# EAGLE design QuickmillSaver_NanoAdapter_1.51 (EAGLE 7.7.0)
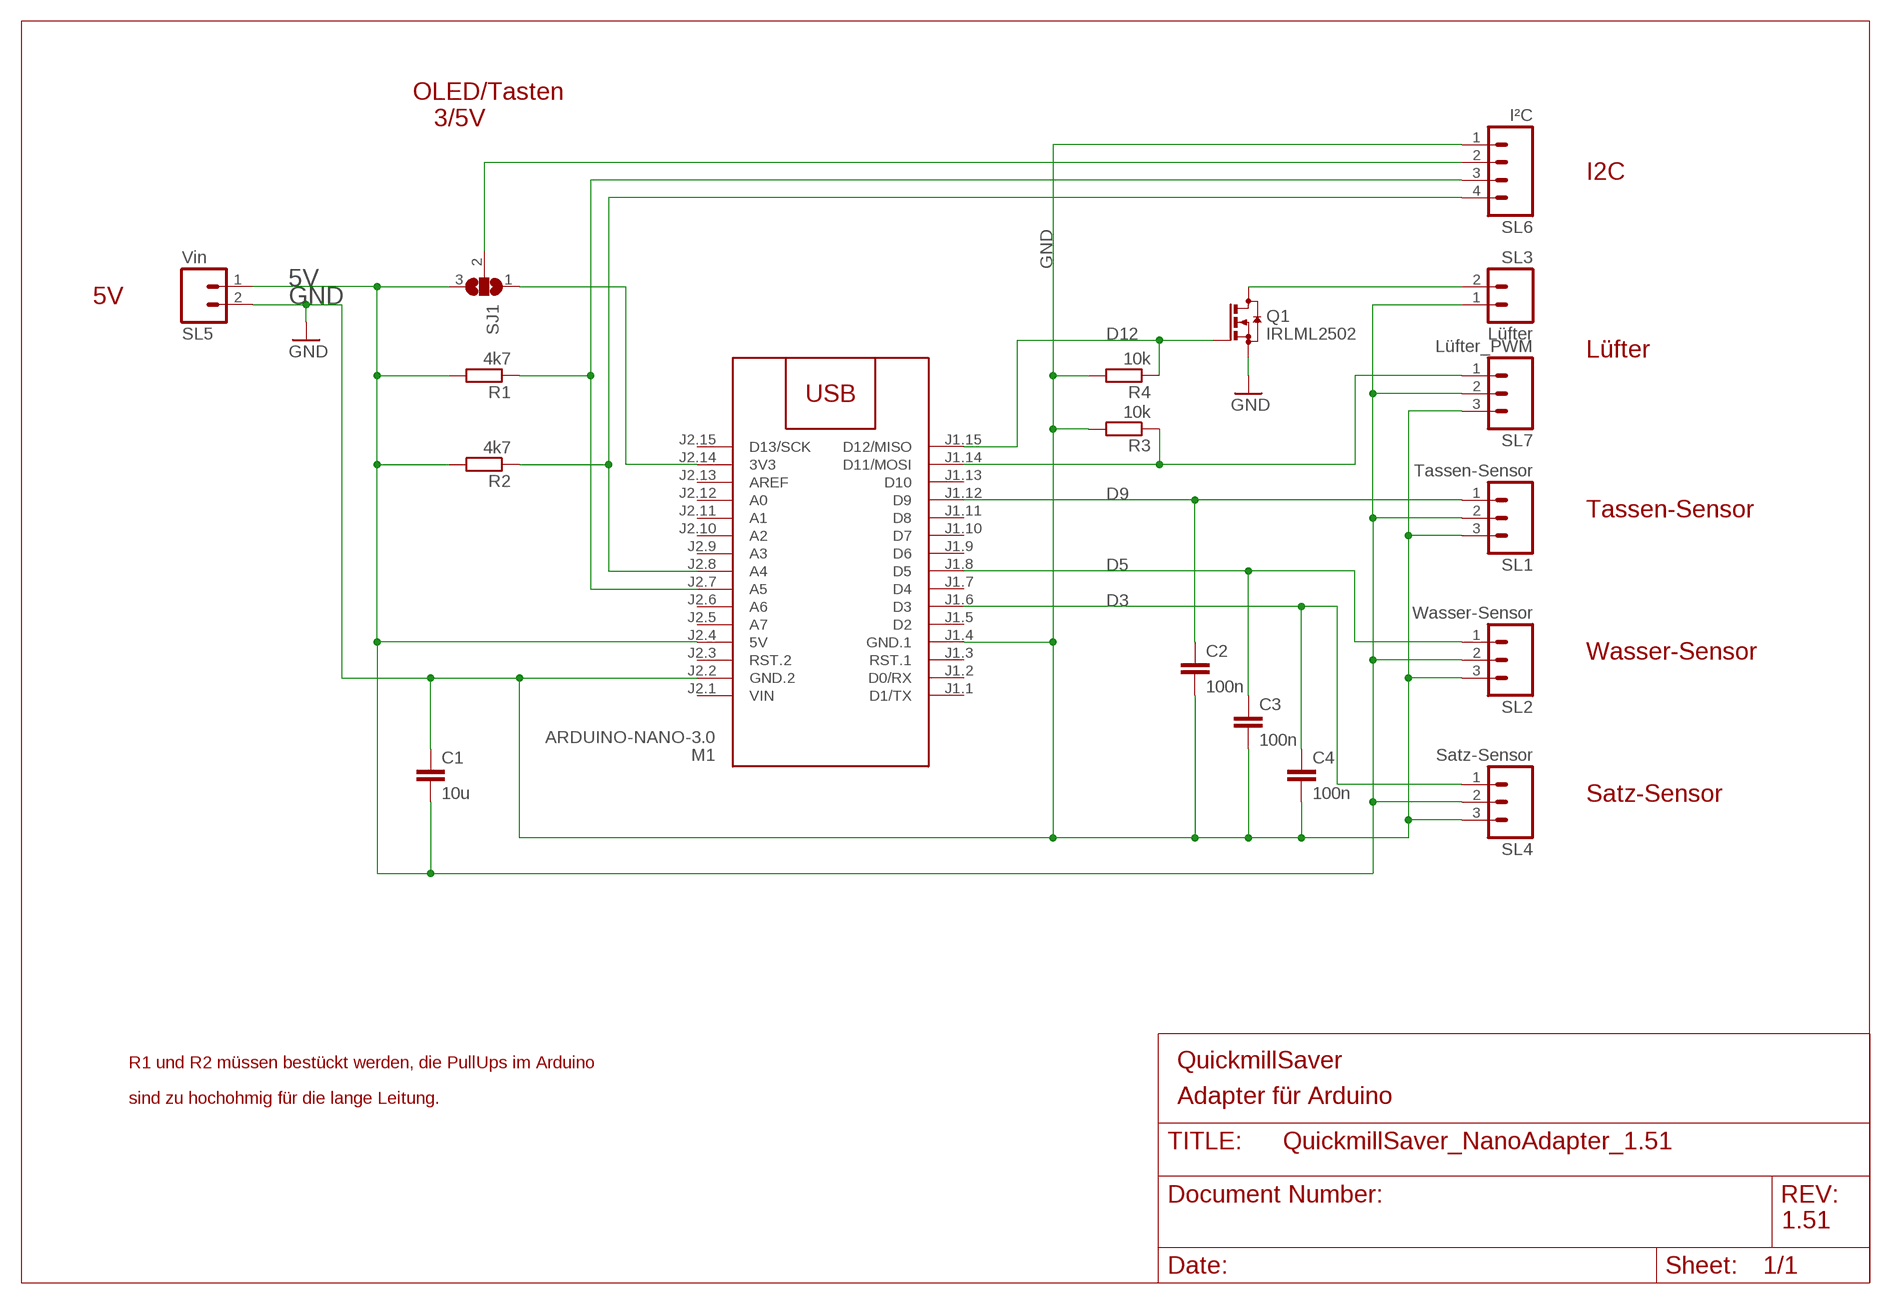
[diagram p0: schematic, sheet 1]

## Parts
C1  10u  C-EUC0805  [C0805]
C2  100n  C-EUC0603  [C0603]
C3  100n  C-EUC0603  [C0603]
C4  100n  C-EUC0603  [C0603]
M1  ARDUINO-NANO-3.0  [ARDUINO-NANO-3.0]
Q1  IRLML2502  BSS123  [SOT23]
R1  4k7  R-EU_R0603  [R0603]
R2  4k7  R-EU_R0603  [R0603]
R3  10k  R-EU_R0603  [R0603]
R4  10k  R-EU_R0603  [R0603]
SJ1  SJ2WW  [SJ_2W]
SL1  Tassen-Sensor  M03  [03P]
SL2  Wasser-Sensor  M03  [03P]
SL3  Lüfter  M02  [02P]
SL4  Satz-Sensor  M03  [03P]
SL5  Vin  M02  [02P]
SL6  I²C  M04  [04P]
SL7  Lüfter_PWM  M03  [03P]

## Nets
5V: C1.2 M1.J2.4(5V) R1.2 R2.2 SJ1.3 SL1.2 SL2.2 SL3.1 SL4.2 SL5.1 SL7.2
D3: C4.1 M1.J1.6(D3) SL4.1
D5: C3.1 M1.J1.8(D5) SL2.1
D9: C2.1 M1.J1.12(D9) SL1.1
D12: M1.J1.15(D12/MISO) Q1.1(G) R4.1
GND: C1.1 C2.2 C3.2 C4.2 M1.J1.4(GND.1) M1.J2.2(GND.2) Q1.2(S) R3.2 R4.2 SL1.3 SL2.3 SL4.3 SL5.2 SL6.1 SL7.3
N$1: M1.J2.14(3V3) SJ1.1
N$2: M1.J1.14(D11/MOSI) R3.1 SL7.1
N$3: Q1.3(D) SL3.2
N$9: SJ1.2 SL6.2
N$10: M1.J2.7(A5) R1.1 SL6.3
N$11: M1.J2.8(A4) R2.1 SL6.4
Unconnected: M1.J1.1(D1/TX) M1.J1.2(D0/RX) M1.J1.3(RST.1) M1.J1.5(D2) M1.J1.7(D4) M1.J1.9(D6) M1.J1.10(D7) M1.J1.11(D8) M1.J1.13(D10) M1.J2.3(RST.2) M1.J2.5(A7) M1.J2.6(A6) M1.J2.9(A3) M1.J2.10(A2) M1.J2.11(A1) M1.J2.12(A0) M1.J2.13(AREF) M1.J2.15(D13/SCK)

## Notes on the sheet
- OLED/Tasten
     3/5V
- I2C
- 5V
- Lüfter
- Tassen-Sensor
- Wasser-Sensor
- Satz-Sensor
- R1 und R2 müssen bestückt werden, die PullUps im Arduino | QuickmillSaver
- sind zu hochohmig für die lange Leitung. | Adapter für Arduino
- 1.51

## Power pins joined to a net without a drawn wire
VIN: M1.J2.1(VIN)

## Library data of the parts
C1-C4 = rcl:C-EU: CAPACITOR, European symbol
M1 = diy-modules:ARDUINO-NANO-3.0: Arduino Nano 3.0 and compatible devices More details available here: https://www.arduino.cc/en/Main/ArduinoBoardNano Click here to find device on ebay.com
Q1 = transistor-small-signal:BSS123: N-CHANNEL MOS FET
R1-R4 = rcl:R-EU_: RESISTOR, European symbol
SJ1 = jumper:SJ2W: SMD solder JUMPER
SL1 SL2 SL4 SL7 = con-amp-quick:M03: AMP QUICK CONNECTOR
SL3 SL5 = con-amp-quick:M02: AMP QUICK CONNECTOR
SL6 = con-amp-quick:M04: AMP QUICK CONNECTOR

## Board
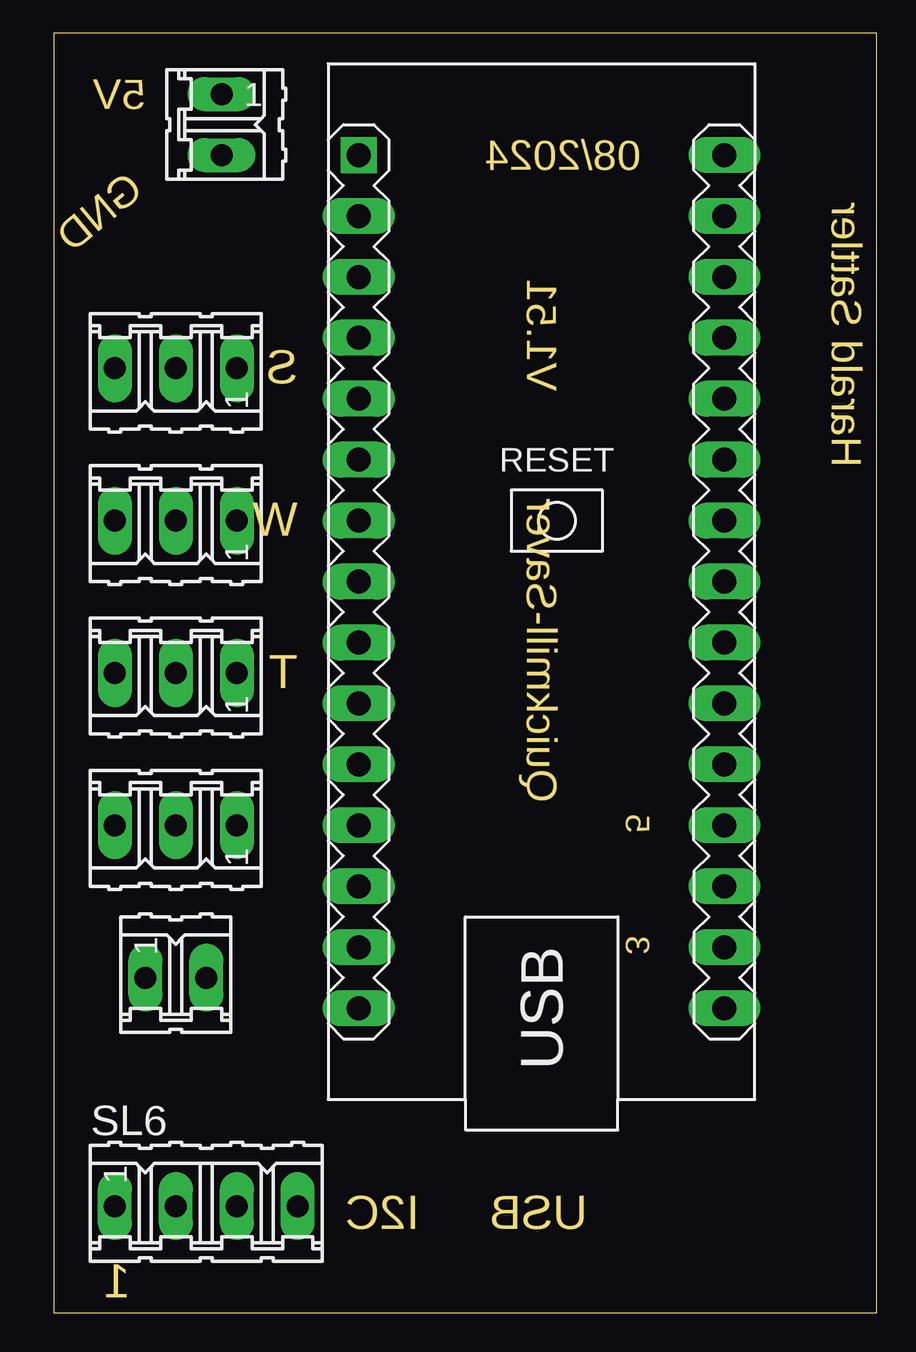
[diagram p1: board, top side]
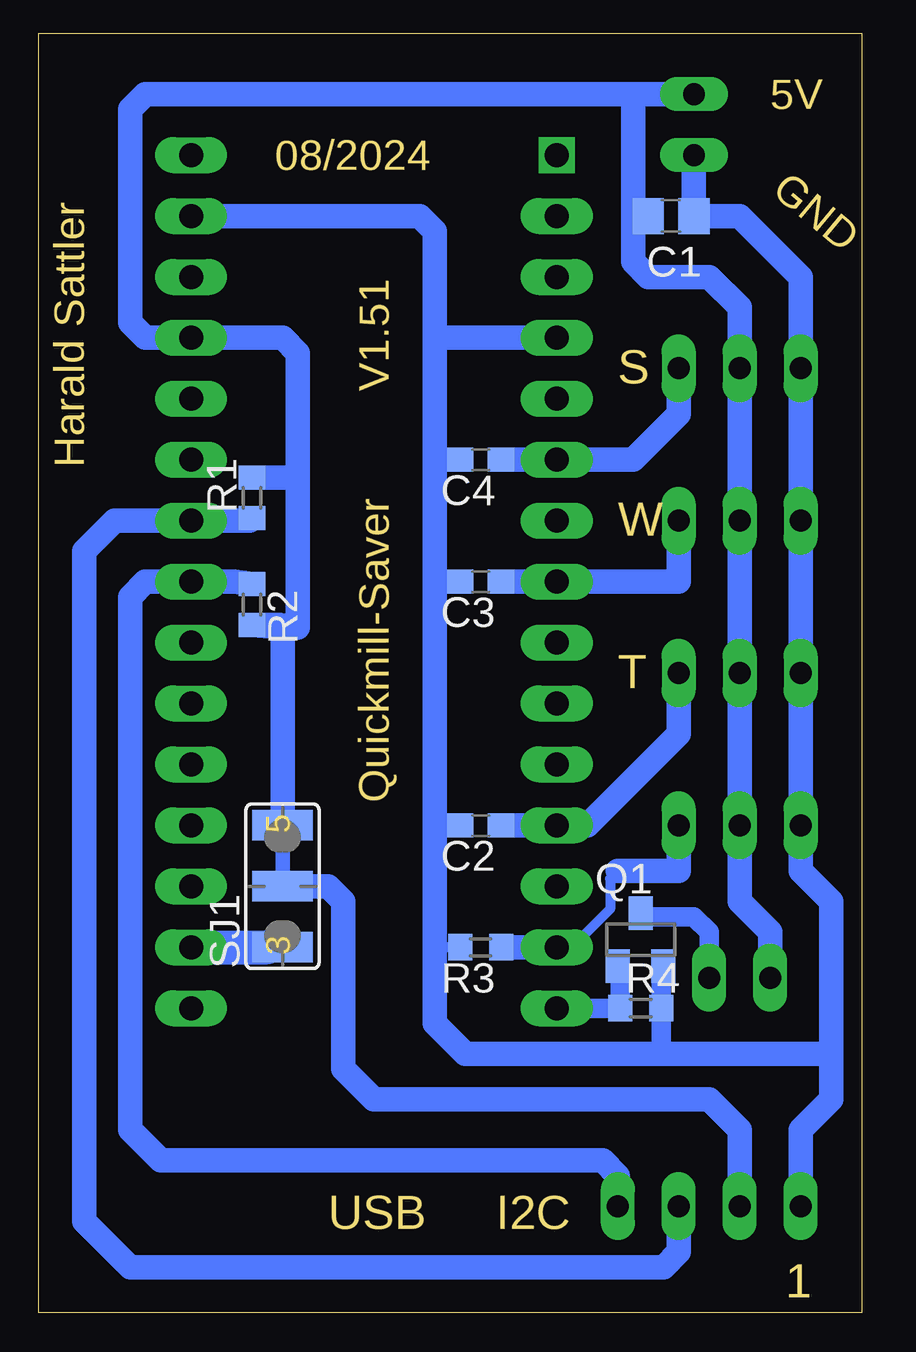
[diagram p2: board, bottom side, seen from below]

No outline drawn. Coordinates in mm, seen from the top.
Copper layers (1*16): Top 0.035mm / dielectric 1.5mm / Bottom 0.035mm
Design rules "default *": minimum track width 10mil, minimum drill 24mil, track to track 0.3mm, track to pad 0.3mm, pad to pad 0.3mm, via to via 0.3mm, smd to smd 0.3mm, copper to edge 40mil, drill to drill 8mil, minimum pad ring 10mil, minimum via ring 8mil, stop-mask expansion 4mil, vias tented up to drill 0mil, thermal gap 10mil
Milling: 4 lines

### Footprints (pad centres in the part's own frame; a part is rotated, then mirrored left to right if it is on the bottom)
C0805 = smd 1.3 x 1.5: 1 -0.95,0; 2 0.95,0
C0603 = smd 1.1 x 1: 1 -0.85,0; 2 0.85,0
ARDUINO-NANO-3.0 = drill 1 pad 1.27 square: J1.1 17.78,7.62 | drill 1 pad 1.27 long: J1.2 15.24,7.62; J1.3 12.7,7.62; J1.4 10.16,7.62; J1.5 7.62,7.62; J1.6 5.08,7.62; J1.7 2.54,7.62; J1.8 0,7.62; J1.9 -2.54,7.62; J1.10 -5.08,7.62; J1.11 -7.62,7.62; J1.12 -10.16,7.62; J1.13 -12.7,7.62; J1.14 -15.24,7.62; J1.15 -17.78,7.62; J2.1 17.78,-7.62; J2.2 15.24,-7.62; J2.3 12.7,-7.62; J2.4 10.16,-7.62; J2.5 7.62,-7.62; J2.6 5.08,-7.62; J2.7 2.54,-7.62; J2.8 0,-7.62; J2.9 -2.54,-7.62; J2.10 -5.08,-7.62; J2.11 -7.62,-7.62; J2.12 -10.16,-7.62; J2.13 -12.7,-7.62; J2.14 -15.24,-7.62; J2.15 -17.78,-7.62
SOT23 = smd 1 x 1.4: 1 -0.95,-1.1; 2 0.95,-1.1; 3 0,1.1
R0603 = smd 1 x 1.1: 1 -0.85,0; 2 0.85,0
SJ_2W = smd 1.27 x 2.54: 1 -2.54,0; 2 0,0; 3 2.54,0
03P = drill 0.914 long: 1 -2.54,0; 2 0,0; 3 2.54,0
02P = drill 0.914 long: 1 -1.27,0; 2 1.27,0
04P = drill 0.914 long: 1 -3.81,0; 2 -1.27,0; 3 1.27,0; 4 3.81,0

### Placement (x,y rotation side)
C1  7.94,45.72 180 bottom
C2  15.88,20.32 180 bottom
C3  15.88,30.48 180 bottom
C4  15.88,35.56 180 bottom
M1  20.32,30.48 90 top
Q1  9.21,15.56 0 bottom
R1  25.4,33.97 90 bottom
R2  25.4,29.53 270 bottom
R3  15.88,15.24 180 bottom
R4  9.21,12.7 0 bottom
SJ1  24.13,17.78 90 bottom
SL1  5.08,26.67 180 top
SL2  5.08,33.02 180 top
SL3  5.08,13.97 0 top
SL4  5.08,39.37 180 top
SL5  6.99,49.53 270 top
SL6  6.35,4.45 0 top
SL7  5.08,20.32 180 top

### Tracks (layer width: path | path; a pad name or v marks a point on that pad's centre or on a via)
5V
  Bottom 0.61: SJ1.3 24.13,17.78
  Bottom 1.016: 23.5,34.92 23.5,40.01 24.13,40.64 M1.J2.4 29.84,40.64 30.48,41.27 30.48,50.16 29.84,50.8 9.53,50.8 | 23.5,34.92 23.5,28.57 24.23,28.68 R2.2 24.13,28.57 SJ1.3 | R1.2 23.6,34.82 23.5,34.92 | SL5.1 9.53,50.8 | 9.53,45.72 9.53,43.81 8.89,43.18 6.35,43.18 5.08,41.91 SL4.2 SL2.2 SL1.2 SL7.2 5.08,17.14 3.81,15.88 SL3.1 | 9.53,45.72 9.53,50.8 | C1.2 9.53,45.72
D3
  Bottom 1.016: SL4.1 7.62,37.47 9.53,35.56 M1.J1.6 C4.1
D5
  Bottom 1.016: SL2.1 7.62,30.48 M1.J1.8 C3.1
D9
  Bottom 1.016: SL1.1 7.62,24.13 11.43,20.32 M1.J1.12 C2.1
D12
  Bottom 0.813: Q1.1 10.06,14.46 R4.1 M1.J1.15
GND
  Bottom 0.406: R3.2 17.78,15.24
  Bottom 0.813: 8.36,14.46 Q1.2 8.36,14.36 R4.2 8.36,10.9 8.26,10.79
  Bottom 1.016: 17.78,40.64 17.78,45.09 18.41,45.72 M1.J2.2 | SL5.2 C1.1 | SL6.1 2.54,7.62 1.27,8.89 1.27,10.79 | 1.27,10.79 1.27,17.14 2.54,18.41 SL7.3 SL1.3 SL2.3 SL4.3 2.54,43.18 5.08,45.72 C1.1 | M1.J1.4 17.78,40.64 | 17.78,40.64 17.78,35.56 | 17.78,35.56 17.78,30.48 | 17.78,30.48 17.78,20.32 | 17.78,20.32 17.78,15.24 17.78,12.06 16.51,10.79 8.26,10.79 1.27,10.79 | C3.2 17.78,30.48 | C4.2 17.78,35.56 | C2.2 17.78,20.32 | C1.1
N$1
  Bottom 1.016: 24.77,15.24 SJ1.1
  Bottom 1.422: M1.J2.14 24.77,15.24
N$2
  Bottom 0.406: 10.16,18.41 10.48,18.1 10.48,16.83 11.75,15.56 12.38,15.56 M1.J1.14
  Bottom 1.016: R3.1 M1.J1.14 | SL7.1 7.62,18.41 10.16,18.41
N$3
  Bottom 0.813: SL3.2 6.35,15.88 6.99,16.51 9.06,16.51 Q1.3
N$9
  Bottom 1.016: SL6.2 5.08,7.62 6.35,8.89 20.32,8.89 21.59,10.16 21.59,17.14 22.23,17.78 SJ1.2
N$10
  Bottom 1.016: R1.1 25.5,33.02 M1.J2.7 31.11,33.02 32.38,31.75 32.38,3.81 30.48,1.91 8.26,1.91 7.62,2.54 SL6.3
N$11
  Bottom 1.016: R2.1 26.14,30.48 M1.J2.8 29.84,30.48 30.48,29.84 30.48,7.62 29.21,6.35 10.79,6.35 10.16,5.71 SL6.4

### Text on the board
Milling: 5V | 08/2024 | GND | S | V1.51 | Harald Sattler | W | T | Quickmill-Saver | 5 | 3 | I2C | USB | 1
